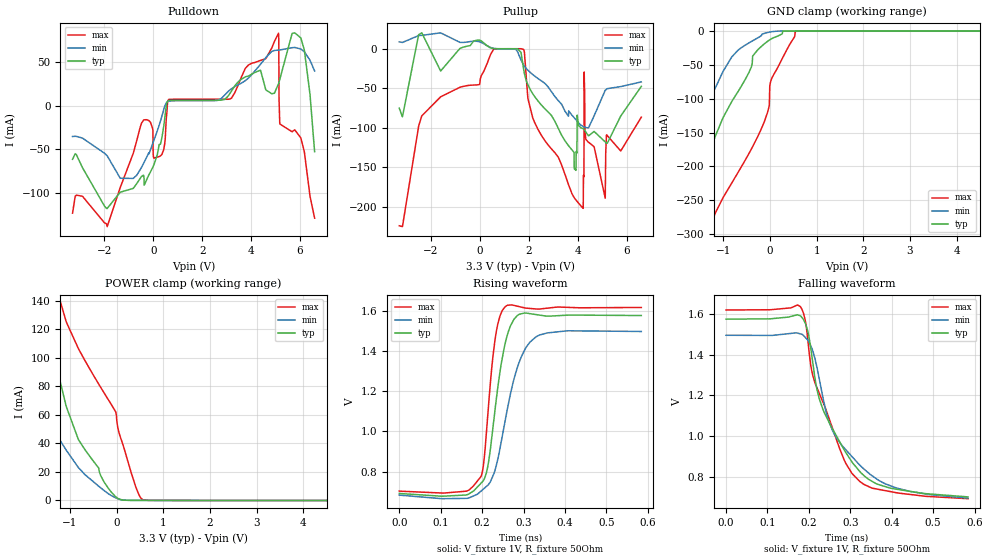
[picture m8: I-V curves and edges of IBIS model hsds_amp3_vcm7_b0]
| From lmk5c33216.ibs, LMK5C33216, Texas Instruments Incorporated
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[Model]   hsds_amp3_vcm7_b0
Model_type   Output
Polarity   Non-Inverting
Vmeas = 1.15
Vref = 1
Cref = 0pF
Rref = 50
|   typ   min   max
C_comp   0.65pF   0.575pF   0.725pF
[Voltage Range]   3.3   3.135   3.465
[Temperature Range]   50   135   -40
[Pullup Reference]   3.3   3.135   3.465
[Pulldown Reference]   -0   0   0
[Power Clamp Reference]   3.3   3.135   3.465
[GND Clamp Reference]   0   0   0
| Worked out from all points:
|   slope of the pulldown table from 0 to 0.495 V, typ, clamps not added: 8.15 ohm
|   slope of the pullup table from 0 to 0.495 V, typ, clamps not added: 49.1 ohm
|   falling waveform, V_fixture 1V, R_fixture 50Ohm: 20-80 % time 96.4ps typ, 104ps min, 87ps max; typ from 1.57 V to 0.702 V
|   rising waveform, V_fixture 1V, R_fixture 50Ohm: 20-80 % time 34.8ps typ, 51.7ps min, 23.8ps max; typ from 0.691 V to 1.58 V
[Pulldown]
|   Voltage   I(typ)   I(min)   I(max)
-3.3V     -61.4mA    -35.32mA   -123.1mA
-1.884V   -117.8mA   -57.35mA   -138.5mA
-815.1mV  -94.71mA   -83.33mA   -54.45mA
-290.4mV  -86.18mA   -60.28mA   -16.06mA
353.1mV   -36.8mA    -12.08mA   -55.92mA
600.6mV   5.448mA    4.845mA    5.51mA
3.165V    15.16mA    18.65mA    7.924mA
5.125V    25.1mA     63.67mA    83.02mA
5.145V    26.92mA    63.73mA    7.956mA
5.184V    31mA       63.85mA    -21.1mA
6.036V    77.63mA    64.95mA    -36.85mA
6.6V      -52.78mA   39.76mA    -128.8mA
[GND Clamp]
|   Voltage   I(typ)   I(min)   I(max)
-3.3V     -892.9mA   -765.6mA   -1.068A
-1.924V   -314.6mA   -288.5mA   -459.9mA
-1.815V   -287mA     -251.4mA   -425.6mA
-1.478V   -218.2mA   -143.5mA   -333.1mA
-1.162V   -154.3mA   -82.94mA   -268mA
-815.1mV  -104mA     -38.12mA   -224.4mA
-171.6mV  -22.09mA   -4.573mA   -142.5mA
-13.2mV   -13.46mA   -1.685mA   -109.6mA
-3.3mV    -13.01mA   -1.546mA   -81.32mA
26.4mV    -11.77mA   -1.169mA   -72.35mA
551.1mV   0A         -83.65nA   -743.3uA
6.6V      0A         0A         0A
[Pullup]
|   Voltage   I(typ)   I(min)   I(max)
-3.3V     -75.08mA   8.679mA    -223.7mA
-2.379V   20.1mA     16.89mA    -84.82mA
570.9mV   83.34uA    399uA      -424.6uA
1.789V    -26.11mA   -20.56mA   -1.218mA
3.858V    -151.9mA   -87.3mA    -188.2mA
4.224V    -101.2mA   -98.24mA   -201.7mA
4.254V    -101.9mA   -98.66mA   -161.9mA
4.264V    -102.2mA   -98.79mA   -29.4mA
4.323V    -105mA     -99.53mA   -112.9mA
5.125V    -117.8mA   -52.44mA   -188.9mA
5.174V    -119.4mA   -51.27mA   -109.1mA
6.6V      -47.56mA   -41.91mA   -86.44mA
[POWER Clamp]
|   Voltage   I(typ)   I(min)   I(max)
-3.3V     330.7mA    180mA      566.4mA
-2.736V   200mA      135.8mA    401.6mA
-1.647V   138.3mA    65.17mA    197.7mA
-1.459V   117.6mA    55.06mA    168.7mA
-1.082V   66.76mA    35.64mA    126mA
-815.1mV  42.67mA    23.06mA    106.5mA
-3.3mV    2.23mA     1.644mA    59.85mA
46.2mV    1.16mA     1.045mA    48.48mA
313.5mV   86.42uA    94.45uA    19.62mA
491.7mV   74.41uA    72.76uA    3.272mA
570.9mV   69.96uA    68.47uA    464.2uA
6.6V      0A         0A         0A
[Ramp]
R_load = 50
|   typ   min   max
dV/dt_r   0.532744/3.46739e-11   0.489978/5.16526e-11   0.549947/2.37434e-11
dV/dt_f   0.523101/9.61309e-11   0.479253/1.04143e-10   0.555318/8.69906e-11
[Falling Waveform]
V_fixture = 1V
V_fixture_min = 0.95V
V_fixture_max = 1.05V
R_fixture = 50Ohm
C_fixture = 0F
|   Time   V(typ)   V(min)   V(max)
0s        1.574V     1.495V     1.619V
179.4ps   1.591V     1.502V     1.636V
192.2ps   1.55V      1.483V     1.558V
208.3ps   1.379V     1.426V     1.309V
233.7ps   1.133V     1.193V     1.169V
260.5ps   1.024V     1.014V     1.019V
289.2ps   919.8mV    933.6mV    867.1mV
322.1ps   829.1mV    860mV      779.7mV
410ps     740.6mV    747mV      723.3mV
584.1ps   702.4mV    696.4mV    693.6mV
[Rising Waveform]
V_fixture = 1V
V_fixture_min = 0.95V
V_fixture_max = 1.05V
R_fixture = 50Ohm
C_fixture = 0F
|   Time   V(typ)   V(min)   V(max)
0s        690.7mV    682.5mV    702.3mV
162.6ps   683.9mV    666.3mV    702.3mV
196.6ps   740.5mV    701.2mV    773.5mV
204.7ps   761.2mV    715.7mV    859.1mV
213.9ps   828.4mV    732.3mV    1.088V
230.9ps   1.104V     805.6mV    1.454V
255.5ps   1.438V     1.053V     1.622V
289ps     1.584V     1.344V     1.623V
328.9ps   1.584V     1.471V     1.612V
584.1ps   1.579V     1.499V     1.619V
